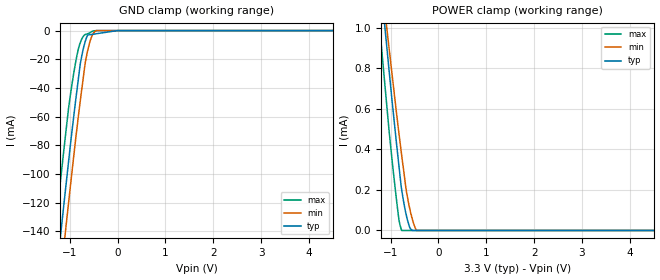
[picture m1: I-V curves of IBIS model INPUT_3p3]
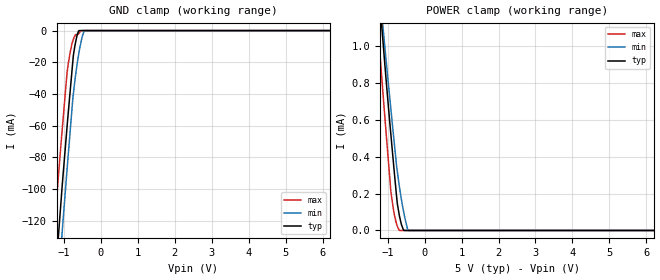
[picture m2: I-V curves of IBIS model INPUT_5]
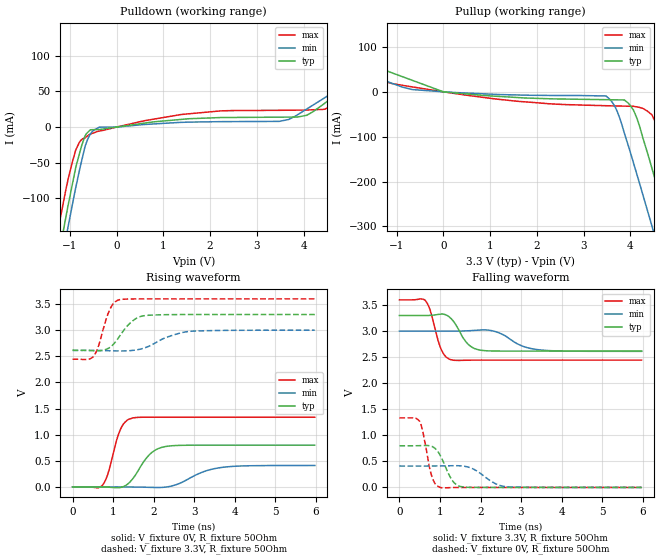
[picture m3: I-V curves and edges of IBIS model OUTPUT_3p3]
|Texas Instruments Incorporated
| 16-Channel LED Driver w/DOT Correction
| Marketing part#   Digital Voltage Range   Package-type   #pins
| TLC5922DAP   3.0v - 5.5v   HTSSOP   32
| TLC5922DAPG4   3.0v - 5.5v   HTSSOP   32
| TLC5922DAPR   3.0v - 5.5v   HTSSOP   32
| TLC5922DAPRG4   3.0v - 5.5v   HTSSOP   32
[IBIS Ver]   3.2
[File name]   tlc5922.ibs
|SIMDE Ver   V2.1 - 201006 - RHL4 - Build 390
[File Rev]   1.0
[Date]   9/23/2010
[Source]
| Texas Instruments Incorporated.
| Analog-eLab Design Center, HPA
| 12500 TI Blvd
| Dallas, TX -75243
| e-mail: elab_ibis@list.ti.com
| -Model generated from simulations in TISPICE
[Notes]   Revision History:
| Rev 1.0: 9/23/2010
| - Initial version of the model
| - Model generated from simulations in TISPICE
| - Model matched to SPICE simulation
| - C_comp although listed in numerical order of value are
|   obtained from varying PVT conditions. For PVT conditions for
|   each specific value refer the buffer description under
|   respective [Model]. IBIS model user is responsible for using
|   appropriate C_comp to simulate for Signal Integrity.
[Disclaimer]
| This model is designed as an aid for customers of Texas Instruments.
| TI and its licensors and suppliers make no warranties, either expressed
| or implied, with respect to this  model, including the warranties of
| merchantability or fitness for a particular purpose. The model is
| provided solely on an "as is" basis. The entire risk as to its quality
| and performance is with the customer.
[Copyright]
 (C) Copyright 2010 Texas Instruments Incorporated.All rights reserved.
|   TLC5922
[Component]   TLC5922
[Manufacturer]   TI
[Package]   |32 HTSSOP -  DAP package
|   typ   min   max
R_pkg   0.07287   0.06337   0.08512
L_pkg   3.05319nH   2.33828nH   4.08640nH
C_pkg   0.51971pF   0.38845pF   0.72323pF
[Pin]  signal_name   model_name   R_pin   L_pin   C_pin
1   GND   GND   0.06913   3.96652nH  0.71298pF
2   BLANK   INPUT   0.06649   3.48030nH  0.69253pF
3   XLAT   INPUT   0.07059   3.22867nH  0.61887pF
4   SCLK   INPUT   0.08104   3.23594nH  0.54000pF
5   SIN   INPUT   0.08466   2.98135nH  0.42389pF
6   PGND   GND   0.00405   0.87852nH  0.27034pF
7   OUT0   TERM   0.06680   2.43622nH  0.38930pF
8   OUT1   TERM   0.06337   2.33828nH  0.38846pF
9   PGND   GND   0.06373   2.35087nH  0.39183pF
10   OUT2   TERM   0.06886   2.50163nH  0.40070pF
11   OUT3   TERM   0.07602   2.73738nH  0.41378pF
12   OUT4   TERM   0.08512   3.00511nH  0.42901pF
13   OUT5   TERM   0.07916   3.26160nH  0.53871pF
14   PGND   GND   0.07130   3.31021nH  0.64105pF
15   OUT6   TERM   0.06727   3.55646nH  0.69695pF
16   OUT7   TERM   0.06994   4.08640nH  0.72323pF
17   OUT8   TERM   0.06904   3.97678nH  0.71219pF
18   OUT9   TERM   0.06643   3.49112nH  0.69180pF
19   PGND   GND   0.07049   3.23862nH  0.61940pF
20   OUT10   TERM   0.07920   3.19571nH  0.53539pF
21   OUT11   TERM   0.08512   3.00537nH  0.43034pF
22   OUT12   TERM   0.07602   2.73753nH  0.41376pF
23   OUT13   TERM   0.06886   2.50182nH  0.40063pF
24   PGND   GND   0.06373   2.35094nH  0.39180pF
25   OUT14   TERM   0.06337   2.33834nH  0.38845pF
26   OUT15   TERM   0.06680   2.43622nH  0.38930pF
27   PGND   GND   0.00405   0.87853nH  0.27032pF
28   SOUT   OUTPUT   0.08466   2.98109nH  0.42395pF
29   NC   NC   0.08105   3.23719nH  0.53982pF
30   MODE   INPUT   0.07059   3.22906nH  0.61913pF
31   IREF   TERM   0.06650   3.48092nH  0.69295pF
32   VCC   POWER   0.06914   3.96756nH  0.71321pF
|   Model Selectors
[Model Selector] INPUT
INPUT_3p3   3.3V digital input
INPUT_5   5.0V digital input
|NOTES   Model INPUT split into three Models INPUT_3p3 and INPUT_5
|   to accomodate vast voltage range of 3.0 V - 5.5V
|   INPUT_3p3 operates in voltage range of 3.0 - 3.3 - 3.6
|   INPUT_5 operates in voltage range of 4.5 - 5.0 - 5.5
|   The max pin frequency for Model INPUT is 30 MHz
|   This is referenced with datasheet
[Model Selector] OUTPUT
OUTPUT_3p3   3.3V digital output
OUTPUT_5   5.0V digital output
|NOTES   Model OUTPUT split into three Models OUTPUT_3p3 and OUTPUT_5
|   to accomodate vast voltage range of 3.0 V - 5.5V
|   OUTPUT_3p3 operates in voltage range of 3.0 - 3.3 - 3.6
|   OUTPUT_5 operates in voltage range of 4.5 - 5.0 - 5.5
|   The min pin frequency for Model OUTPUT is 15 MHz
|   This is referenced with datasheet
[Model Selector] TERM
TERM_3p3  3.3V nominal termination
TERM_5   5.0V nominal termination
[Model]  TERM_3p3
Model_type Terminator
C_comp   1.0e-20F  1.0e-20F  1.0e-20F
|   typ   min   max
[Voltage Range]   3.3V   3.0V   3.6V
[POWER Clamp Reference]   3.3V   3.0V   3.6V
[GND Clamp Reference]   0V   0V   0V
|Ambient Temperature   25   85   -20
|Junction Temperature
[Temperature Range]   65   125   -20
[Model]  TERM_5
Model_type Terminator
C_comp   1.0e-20F  1.0e-20F  1.0e-20F
|   typ   min   max
[Voltage Range]   5.0V   4.5V   5.5V
[POWER Clamp Reference]   5.0V   4.5V   5.5V
[GND Clamp Reference]   0V   0V   0V
|Ambient Temperature   25   85   -20
|Junction Temperature
[Temperature Range]   65   125   -20
| Models and submodels in the file (6): INPUT_3p3 (Input), INPUT_5 (Input), OUTPUT_3p3 (Output), OUTPUT_5 (Output), TERM_3p3 (Terminator), TERM_5 (Terminator)
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|   input_3p3 Model
[Model]   INPUT_3p3
Model_type   Input
Vinl = 0.66
Vinh = 2.64
|   typ   min   max
|   (nom PVT)   (Fast PVT)   (slow PVT)
|Average
C_comp   1.234e-12   1.233e-12   1.250e-12
| Where nom  PVT is Nominal Process,  3.3V,  65C
|   Fast PVT is Strong Process,   3.6V,  -20C
|   Slow PVT is Weak Process,   3V,  125C
[Model Spec]
Vinl   0.66   0.6   0.72
Vinh   2.64   2.4   2.88
[Voltage Range]   3.3   3   3.6
|Ambient Temperature   25   85   -20
|Junction Temperature
[Temperature Range]   65   125   -20
[Power Clamp Reference]   3.3   3   3.6
[GND Clamp Reference]   0   0   0
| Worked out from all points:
|   GND clamp passes 1 mA (typ) near -0.20 V on its own axis
|   POWER clamp passes 1 mA (typ) near -1.12 V on its own axis
[GND Clamp]
|   Voltage   I(typ)   I(min)   I(max)
-3.3V     -833.7mA   -861.1mA   -796.6mA
-1.353V   -194mA     -223.3mA   -155mA
-1.263V   -165.5mA   -194.6mA   -126.5mA
-1.178V   -138.6mA   -167.9mA   -100.2mA
-1.086V   -110.2mA   -139.1mA   -72.37mA
-1.025V   -91.6mA    -120.4mA   -54.34mA
-913.2mV  -59.09mA   -86.8mA    -29.1mA
-778.8mV  -23.14mA   -48.95mA   -8.409mA
-643.5mV  -4.396mA   -16.97mA   -2.387mA
-546mV    -2.705mA   -4.622mA   -795.3uA
-447mV    -2.215mA   0A         -23.82uA
6.6V      0A         0A         0A
[POWER Clamp]
|   Voltage   I(typ)   I(min)   I(max)
-3.3V     6.641mA    5.924mA    6.756mA
-1.223V   1.261mA    1.305mA    990.3uA
-1.122V   1.01mA     1.089mA    725.7uA
-1.068V   878.1uA    974.5uA    586uA
-963.6mV  626.7uA    758.8uA    334.9uA
-870mV    414.9uA    565.6uA    137.9uA
-823.2mV  313.4uA    475.8uA    48.83uA
-769.2mV  202.8uA    372.8uA    0A
-675mV    78.81uA    201.6uA    0A
-607.2mV  18.87uA    116.3uA    0A
-459mV    0A         0A         0A
6.6V      0A         0A         0A
|   input_5 Model
[Model]   INPUT_5
Model_type   Input
Vinl = 1
Vinh = 4
|   typ   min   max
|   (nom PVT)   (Fast PVT)   (slow PVT)
|Average
C_comp   1.272e-12   1.155e-12   1.312e-12
| Where nom  PVT is Nominal Process,  5V,  65C
|   Fast PVT is Strong Process,   5.5V,  -20C
|   Slow PVT is Weak Process,   4.5V,  125C
[Model Spec]
Vinl   1   0.9   1.1
Vinh   4   3.6   4.4
[Voltage Range]   5   4.5   5.5
|Ambient Temperature   25   85   -20
|Junction Temperature
[Temperature Range]   65   125   -20
[Power Clamp Reference]   5   4.5   5.5
[GND Clamp Reference]   0   0   0
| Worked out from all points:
|   GND clamp passes 1 mA (typ) near -0.62 V on its own axis
|   POWER clamp passes 1 mA (typ) near -1.12 V on its own axis
[GND Clamp]
|   Voltage   I(typ)   I(min)   I(max)
-5V       -1.4A      -1.426A    -1.364A
-1.288V   -173.4mA   -202.5mA   -134.3mA
-1.205V   -147.3mA   -176.7mA   -108.4mA
-1.079V   -107.9mA   -137.1mA   -71.48mA
-1.045V   -97.46mA   -126.6mA   -62.24mA
-913.5mV  -60.24mA   -87.37mA   -26.32mA
-831mV    -38.31mA   -63.6mA    -13.71mA
-745mV    -15.88mA   -40.05mA   -5.57mA
-650mV    -3.618mA   -22.37mA   -2.466mA
-590mV    0A         -13.38mA   -1.609mA
-450.5mV  0A         0A         0A
10V       0A         0A         0A
[POWER Clamp]
|   Voltage   I(typ)   I(min)   I(max)
-5V       11.11mA    9.763mA    11.54mA
-1.345V   1.567mA    1.569mA    1.322mA
-1.224V   1.265mA    1.309mA    997.3uA
-1.183V   1.162mA    1.22mA     886.2uA
-1.051V   835.8uA    939.4uA    549.7uA
-913.5mV  520uA      657.8uA    211.3uA
-820mV    313.9uA    470.5uA    87.32uA
-740mV    147.2uA    321uA      23.81uA
-680mV    76.91uA    233.8uA    112nA
-570mV    1.458uA    103.8uA    0A
-450.5mV  0A         0A         0A
10V       0A         0A         0A
|   output_3p3 Model
[Model]   OUTPUT_3p3
Model_type   Output
Polarity   Non-Inverting
Vmeas = 1.65
Vref = 1.65
Cref = 15pF
Rref = 50
|   typ   min   max
|   (nom PVT)   (Fast PVT)   (slow PVT)
C_comp   1.884e-12   1.787e-12   1.943e-12
|ON state : BUFFER OUTPUT TURNED HIGH
|C_comp   1.884e-12   1.787e-12   1.943e-12
|OFF state: BUFFER OUTPUT TURNED LOW
|C_comp   1.657e-12   1.637e-12   1.681e-12
| Where nom  PVT is Nominal Process,  3.3V,  65C
|   Fast PVT is Strong Process,   3.6V,  -20C
|   Slow PVT is Weak Process,   3V,  125C
[Voltage Range]   3.3   3   3.6
|Ambient Temperature   25   85   -20
|Junction Temperature
[Temperature Range]   65   125   -20
[Pullup Reference]   3.3   3   3.6
[Pulldown Reference]   0   0   0
[Power Clamp Reference]   3.3   3   3.6
[GND Clamp Reference]   0   0   0
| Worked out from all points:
|   slope of the pulldown table from 0 to 0.495 V, typ, clamps not added: 108 ohm
|   slope of the pullup table from 0 to 0.495 V, typ, clamps not added: 104 ohm
|   falling waveform, V_fixture 3.3V, R_fixture 50Ohm: 20-80 % time 333ps typ, 544ps min, 246ps max; typ from 3.3 V to 2.62 V
|   rising waveform, V_fixture 0V, R_fixture 50Ohm: 20-80 % time 438ps typ, 705ps min, 285ps max; typ from 0 V to 0.8 V
|   rising waveform, V_fixture 3.3V, R_fixture 50Ohm: 20-80 % time 426ps typ, 677ps min, 273ps max; typ from 2.62 V to 3.3 V
|   falling waveform, V_fixture 0V, R_fixture 50Ohm: 20-80 % time 294ps typ, 463ps min, 201ps max; typ from 0.8 V to 0 V
[Pulldown]
|   Voltage   I(typ)   I(min)   I(max)
-3.3V     -954.6mA   -968.7mA   -931.5mA
-1.262V   -189.9mA   -219.1mA   -148.8mA
-1.131V   -143mA     -172.7mA   -103.7mA
-1.043V   -112mA     -142.1mA   -75.28mA
-873.6mV  -57.07mA   -85.2mA    -32.49mA
-749.1mV  -26.68mA   -48.05mA   -17.76mA
-498mV    -3.662mA   -4.783mA   -8.385mA
1.38V     10.73mA    6.593mA    17.6mA
3.48V     13.9mA     7.977mA    23.53mA
4.066V    16.52mA    25.19mA    23.9mA
4.573V    39.24mA    46.36mA    29.4mA
6.6V      141.7mA    134.6mA    148.3mA
[Pullup]
|   Voltage   I(typ)   I(min)   I(max)
-3.3V     127mA      112.9mA    141.2mA
-1.104V   42.48mA    19.06mA    18.5mA
0V        0A         0A         0A
3.48V     -17.51mA   -9.231mA   -31mA
3.678V    -17.82mA   -34.46mA   -31.46mA
3.871V    -18.13mA   -92.12mA   -31.84mA
4.138V    -58.33mA   -183.6mA   -33.58mA
4.458V    -169.3mA   -297.9mA   -51.09mA
4.584V    -215.2mA   -343.6mA   -81.43mA
4.793V    -291.6mA   -420.1mA   -153.5mA
5.184V    -437.6mA   -563.9mA   -301.4mA
6.6V      -975mA     -1.091A    -850.3mA
[Ramp]
R_load = 50
|   typ   min   max
dV/dt_r   0.479733/4.37847e-10   0.24657/7.02497e-10   0.800374/2.84515e-10
dV/dt_f   0.409789/3.32963e-10   0.232626/5.40615e-10   0.693219/2.46259e-10
[Falling Waveform]
V_fixture = 3.3V
V_fixture_min = 3V
V_fixture_max = 3.6V
R_fixture = 50Ohm
|   Time   V(typ)   V(min)   V(max)
0s        3.3V       3V         3.6V
625ps     3.3V       3V         3.599V
750ps     3.302V     3V         3.419V
1.025ns   3.326V     3V         2.66V
1.275ns   3.24V      2.999V     2.451V
1.675ns   2.764V     3.006V     2.442V
1.975ns   2.638V     3.02V      2.444V
2.375ns   2.618V     2.989V     2.445V
3.375ns   2.617V     2.649V     2.445V
5.975ns   2.617V     2.612V     2.445V
[Rising Waveform]
V_fixture = 0V
V_fixture_min = 0V
V_fixture_max = 0V
R_fixture = 50Ohm
|   Time   V(typ)   V(min)   V(max)
0s        215pV      1.703nV    197.8pV
750ps     -1.813mV   368.3uV    44.24mV
875ps     -4.92mV    420.4uV    257mV
1.175ns   -11.25mV   67.6uV     1.09V
1.275ns   13.14mV    -365.6uV   1.224V
1.475ns   146.3mV    -1.643mV   1.318V
1.9ns     620.3mV    -7.76mV    1.334V
2.3ns     774.1mV    -2.81mV    1.334V
3.65ns    799.5mV    370.1mV    1.334V
5.975ns   799.6mV    410.9mV    1.334V
[Rising Waveform]
V_fixture = 3.3V
V_fixture_min = 3V
V_fixture_max = 3.6V
R_fixture = 50Ohm
|   Time   V(typ)   V(min)   V(max)
0s        2.617V     2.612V     2.444V
525ps     2.609V     2.612V     2.507V
650ps     2.608V     2.611V     2.72V
900ps     2.661V     2.606V     3.363V
1.025ns   2.745V     2.604V     3.525V
1.15ns    2.873V     2.602V     3.583V
1.5ns     3.189V     2.615V     3.598V
1.825ns   3.283V     2.675V     3.6V
2.9ns     3.3V       2.978V     3.6V
5.975ns   3.3V       3V         3.6V
[Falling Waveform]
V_fixture = 0V
V_fixture_min = 0V
V_fixture_max = 0V
R_fixture = 50Ohm
|   Time   V(typ)   V(min)   V(max)
0s        799.7mV    411.1mV    1.334V
500ps     802.1mV    410.8mV    1.269V
575ps     804.3mV    410.8mV    1.077V
800ps     787.3mV    411.4mV    212.4mV
900ps     732.8mV    412mV      50.07mV
1.025ns   587.4mV    413mV      -3.73mV
1.3ns     138.2mV    416.8mV    -2.336mV
1.575ns   9.088mV    409.4mV    177.3uV
2.625ns   87.69uV    15.16mV    224.9uV
5.975ns   70.5uV     25.93uV    166.5uV
